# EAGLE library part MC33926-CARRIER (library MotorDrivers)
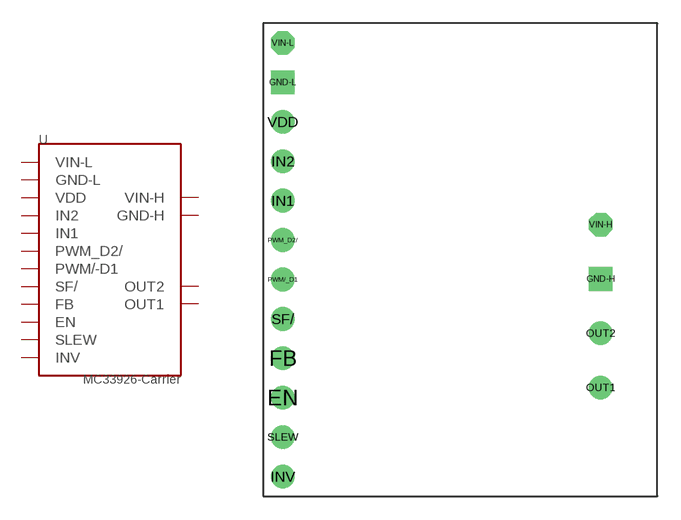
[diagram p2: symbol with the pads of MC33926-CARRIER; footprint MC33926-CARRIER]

Designator prefix -

## MC33926-CARRIER  [MC33926-CARRIER]
EN  EN
FB  FB
GND-H  GND-H
GND-L  GND-L
IN1  IN1
IN2  IN2
INV  INV
OUT1  OUT1
OUT2  OUT2
PWM/_D1  PWM/-D1
PWM_D2/  PWM_D2/
SF/  SF/
SLEW  SLEW
VDD  VDD
VIN-H  VIN-H
VIN-L  VIN-L

## Footprint MC33926-CARRIER (pad centres in mm)
drill 1.016: EN -11.43,-8.89; FB -11.43,-6.35; IN1 -11.43,3.81; IN2 -11.43,6.35; INV -11.43,-13.97; OUT1 9.05,-8.24; OUT2 9.05,-4.74; PWM/_D1 -11.43,-1.27; PWM_D2/ -11.43,1.27; SF/ -11.43,-3.81; SLEW -11.43,-11.43; VDD -11.43,8.89
drill 1.016 square: GND-H 9.05,-1.24; GND-L -11.43,11.43
drill 1.016 octagon: VIN-H 9.05,2.261; VIN-L -11.43,13.97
